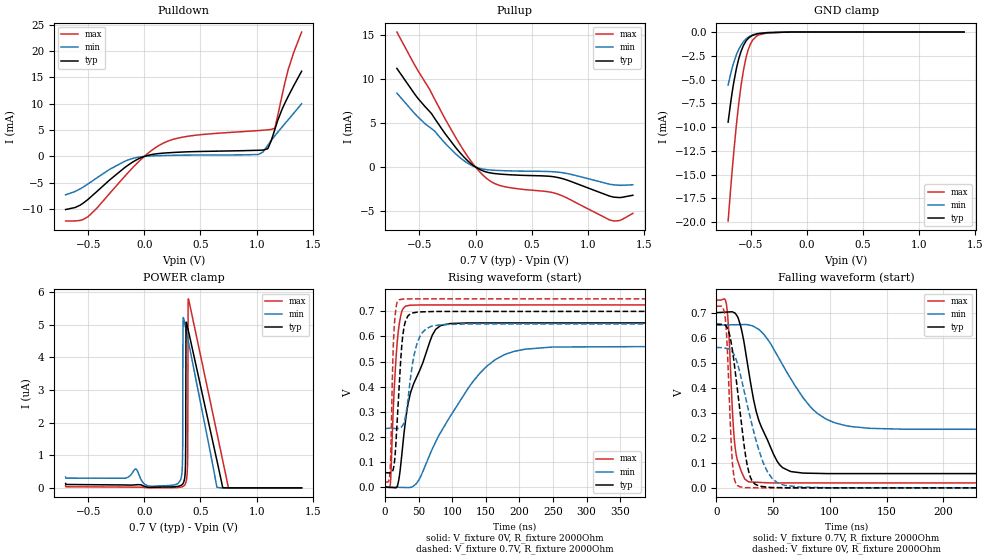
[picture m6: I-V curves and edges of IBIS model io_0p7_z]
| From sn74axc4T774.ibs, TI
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|   io_0p7_z Model
[Model]   io_0p7_z
Model_type   I/O
Polarity   Non-Inverting
Enable   Active-Low
Vinl = 0.21
Vinh = 0.49
Vmeas = 0.35
Vref = 0
Cref = 2pF
Rref = 100000
|   typ   min   max
C_comp   1.843pF   1.651pF   2.136pF
[Model spec]
|subparameter
Vinl   0.21   0.195   0.225
Vinh   0.49   0.455   0.525
| Where Nom  PVT is Nominal Process, 0.7V, 27C
|   Fast PVT is Strong Process,  0.75V, -40C
|   Slow PVT is Weak Process,   0.65V, 130C
[Voltage Range]   0.7   0.65   0.75
|Junction Temperature
[Temperature Range]   27   130   -40
[Pullup Reference]   0.7   0.65   0.75
[Pulldown Reference]   0   -0   0
[Power Clamp Reference]   0.7   0.65   0.75
[GND Clamp Reference]   0   0   0
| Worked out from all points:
|   slope of the pulldown table from 0 to 0.105 V, typ, clamps not added: 215 ohm
|   slope of the pullup table from 0 to 0.105 V, typ, clamps not added: 176 ohm
|   GND clamp passes 1 mA (typ) near -0.54 V on its own axis
|   falling waveform, V_fixture 0.7V, R_fixture 2000Ohm: 20-80 % time 20.8ns typ, 35.4ns min, 5.27ns max; typ from 0.7 V to 0.057 V
|   rising waveform, V_fixture 0V, R_fixture 2000Ohm: 20-80 % time 34.7ns typ, 75.5ns min, 8.28ns max; typ from 0 V to 0.654 V
|   rising waveform, V_fixture 0.7V, R_fixture 2000Ohm: 20-80 % time 8.78ns typ, 14.5ns min, 4.15ns max; typ from 0.057 V to 0.7 V
|   falling waveform, V_fixture 0V, R_fixture 2000Ohm: 20-80 % time 10.7ns typ, 19ns min, 4.1ns max; typ from 0.654 V to 0 V
[Pulldown]
|   Voltage   I(typ)   I(min)   I(max)
-700mV    -10.08mA   -7.288mA   -12.26mA
-500.5mV  -8.149mA   -5.217mA   -11.44mA
-307.3mV  -4.449mA   -2.441mA   -7.001mA
-86.8mV   -856.9uA   -293.1uA   -1.782mA
177.8mV   643.8uA    177.3uA    2.615mA
436.1mV   913.6uA    262.7uA    3.974mA
1.016V    1.174mA    368.7uA    4.912mA
1.058V    1.211mA    889.2uA    4.983mA
1.1V      1.534mA    2.123mA    5.062mA
1.161V    5.052mA    3.892mA    5.373mA
1.278V    11.31mA    6.902mA    16.3mA
1.4V      16.17mA    10mA       23.62mA
[GND Clamp]
|   Voltage   I(typ)   I(min)   I(max)
-700mV    -9.473mA   -5.569mA   -19.87mA
-674.8mV  -7.198mA   -4.264mA   -16.07mA
-649.6mV  -5.285mA   -3.192mA   -12.61mA
-622.3mV  -3.629mA   -2.276mA   -9.304mA
-584.5mV  -2.013mA   -1.371mA   -5.599mA
-544.6mV  -1.015mA   -772.1uA   -2.899mA
-521.5mV  -677.6uA   -547uA     -1.878mA
-481.6mV  -348uA     -300.8uA   -843.7uA
-443.8mV  -200.2uA   -174.6uA   -401uA
-351.4mV  -69.33uA   -55.44uA   -97.88uA
-175mV    -6.308uA   -6.304uA   -6.326uA
1.4V      0A         0A         0A
[Pullup]
|   Voltage   I(typ)   I(min)   I(max)
-700mV    11.23mA    8.411mA    15.37mA
-511mV    7.79mA     5.678mA    10.94mA
-391.3mV  6.072mA    4.371mA    8.404mA
-267.4mV  3.741mA    2.66mA     5.406mA
-145.6mV  1.739mA    1.149mA    2.703mA
-4.9mV    40.88uA    22.8uA     76.51uA
116.9mV   -634.1uA   -323.2uA   -1.476mA
266mV     -849.2uA   -422.9uA   -2.255mA
736.4mV   -1.204mA   -587.7uA   -3.104mA
1.219V    -3.394mA   -2.009mA   -6.11mA
1.291V    -3.469mA   -2.081mA   -6.047mA
1.4V      -3.212mA   -2.026mA   -5.275mA
[POWER Clamp]
|   Voltage   I(typ)   I(min)   I(max)
-700mV    133.1nA    328.6nA    61.75nA
301.7mV   46.58nA    137.2nA    11.38nA
339.5mV   110nA      741.1nA    37.1nA
345.8mV   140.3nA    5.172uA    47.42nA
360.5mV   333.2nA    5.024uA    93.03nA
368.9mV   1.505uA    4.883uA    151.5nA
371mV     4.867uA    4.848uA    174.4nA
385.7mV   4.915uA    4.597uA    910.4nA
389.9mV   4.851uA    4.525uA    5.707uA
392mV     4.819uA    4.489uA    5.794uA
751.1mV   0A         0A         0A
1.4V      0A         0A         0A
[Ramp]
R_load = 2000
|   typ   min   max
dV/dt_r   0.39249/3.48536e-08   0.336587/7.54689e-08   0.435458/8.28278e-09
dV/dt_f   0.385908/2.08278e-08   0.25001/3.52788e-08   0.438177/5.25426e-09
[Falling Waveform]
V_fixture = 0.7V
V_fixture_min = 0.65V
V_fixture_max = 0.75V
R_fixture = 2000Ohm
C_fixture = 0F
|   Time   V(typ)   V(min)   V(max)
0s        700mV      650mV      750mV
8.728ns   702.1mV    650.8mV    737.6mV
10.89ns   702.6mV    651.1mV    629.1mV
16.65ns   697.5mV    651.6mV    158.3mV
28.27ns   472.5mV    651mV      24.52mV
39.54ns   244.6mV    623.9mV    21.35mV
66.2ns    64.69mV    431.3mV    19.73mV
89.26ns   57.74mV    296.6mV    19.73mV
118.4ns   56.96mV    245mV      19.73mV
500ns     56.82mV    233.3mV    19.7mV
[Rising Waveform]
V_fixture = 0V
V_fixture_min = 0V
V_fixture_max = 0V
R_fixture = 2000Ohm
C_fixture = 0F
|   Time   V(typ)   V(min)   V(max)
0s        816.2nV    11.57uV    -213.6nV
7.73ns    -1.656mV   -543.5uV   9.219mV
13.05ns   -2.796mV   -925.4uV   359.5mV
17.91ns   2.087mV    -1.274mV   571.7mV
29.81ns   250.2mV    -2.129mV   719.9mV
38.14ns   378.1mV    -1.126mV   724.7mV
75.32ns   628.3mV    179.7mV    725.7mV
129.8ns   654mV      416.7mV    725.7mV
178.2ns   654mV      528mV      725.7mV
500ns     654.2mV    561mV      725.8mV
[Rising Waveform]
V_fixture = 0.7V
V_fixture_min = 0.65V
V_fixture_max = 0.75V
R_fixture = 2000Ohm
C_fixture = 0F
|   Time   V(typ)   V(min)   V(max)
0s        56.81mV    233.3mV    19.7mV
7.273ns   56.07mV    234.3mV    55.54mV
13.05ns   82.77mV    234mV      611.2mV
16.5ns    191.4mV    232.4mV    717.8mV
20.59ns   382.5mV    234.6mV    745.9mV
26.05ns   596.5mV    245.4mV    749.1mV
30.93ns   665.4mV    289.1mV    749.5mV
46.52ns   696.5mV    562.5mV    750mV
68.85ns   699.3mV    640.8mV    750mV
500ns     700mV      650mV      750mV
[Falling Waveform]
|Gnd
V_fixture = 0V
V_fixture_min = 0V
V_fixture_max = 0V
R_fixture = 2000Ohm
C_fixture = 0F
|   Time   V(typ)   V(min)   V(max)
0s        654.2mV    561mV      725.8mV
7.73ns    650.1mV    558.5mV    682.4mV
9.443ns   640.5mV    556.7mV    577.3mV
14.33ns   544.1mV    542mV      92.13mV
20.59ns   315.9mV    463.8mV    4.219mV
27.1ns    92.9mV     334mV      673.8uV
31.37ns   29.19mV    252.9mV    409.6uV
45.09ns   2.916mV    63.42mV    36.01uV
59.98ns   471.2uV    10.1mV     34.82uV
500ns     826nV      11.58uV    -203.9nV
